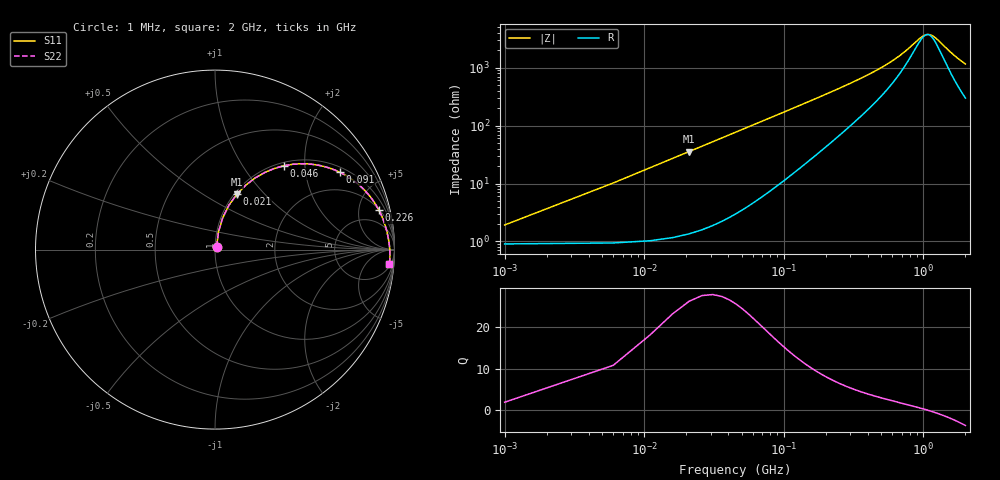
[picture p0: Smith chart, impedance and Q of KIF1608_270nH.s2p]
# MHz S RI R 50
!Freq ReS11 ImS11 ReS21 ImS21 ReS12 ImS12 ReS22 ImS22
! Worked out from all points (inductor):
!   401 points, 1 MHz to 2 GHz, reference 50 ohm
!   read as one part in series: L = 270 nH near 11 MHz
!   highest Q = 26.3 at 21 MHz (marker M1), where L = 270 nH
!   self-resonance near 1.063 GHz
!   S11 on the Smith chart (normalised r, x): 1 MHz: 1.02, +0.03; 21 MHz: 1.03, +0.71; 46 MHz: 1.06, +1.56; 91 MHz: 1.19, +3.10; 226 MHz: 2.10, +7.82; 2 GHz: 7, -22
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1  0.00926 0.0166  0.9907 -0.0166  0.9907 -0.0166  0.00926 0.0166
6  0.0193 0.0988  0.9807 -0.0988  0.9807 -0.0988  0.0193 0.0988
16  0.0778 0.2473  0.9222 -0.2473  0.9222 -0.2473  0.0778 0.2473
21  0.1218 0.3086  0.8782 -0.3086  0.8782 -0.3086  0.1218 0.3086
31  0.2249 0.4  0.7751 -0.4  0.7751 -0.4  0.2249 0.4
46  0.3834 0.467  0.6166 -0.467  0.6166 -0.467  0.3834 0.467
66  0.5548 0.4737  0.4452 -0.4737  0.4452 -0.4737  0.5548 0.4737
91  0.6955 0.4309  0.3045 -0.4309  0.3045 -0.4309  0.6955 0.4309
116  0.7804 0.3784  0.2196 -0.3784  0.2196 -0.3784  0.7804 0.3784
141  0.8332 0.331  0.1668 -0.331  0.1668 -0.331  0.8332 0.331
176  0.8778 0.2772  0.1222 -0.2772  0.1222 -0.2772  0.8778 0.2772
226  0.9125 0.221  0.0875 -0.221  0.0875 -0.221  0.9125 0.221
336  0.9444 0.1463  0.0556 -0.1463  0.0556 -0.1463  0.9444 0.1463
476  0.9592 0.0944  0.0408 -0.0944  0.0408 -0.0944  0.9592 0.0944
671  0.9677 0.0518  0.0323 -0.0518  0.0323 -0.0518  0.9677 0.0518
896  0.9721 0.0192  0.0279 -0.0192  0.0279 -0.0192  0.9721 0.0192
1001  0.9733 0.00681  0.0267 -0.00681  0.0267 -0.00681  0.9733 0.00681
1066  0.9739 -0.000283  0.0261 0.000283  0.0261 0.000283  0.9739 -0.000283
1136  0.9743 -0.00753  0.0257 0.00753  0.0257 0.00753  0.9743 -0.00753
1336  0.9749 -0.0265  0.0251 0.0265  0.0251 0.0265  0.9749 -0.0265
1671  0.9741 -0.0546  0.0259 0.0546  0.0259 0.0546  0.9741 -0.0546
2000  0.9717 -0.0794  0.0283 0.0794  0.0283 0.0794  0.9717 -0.0794
